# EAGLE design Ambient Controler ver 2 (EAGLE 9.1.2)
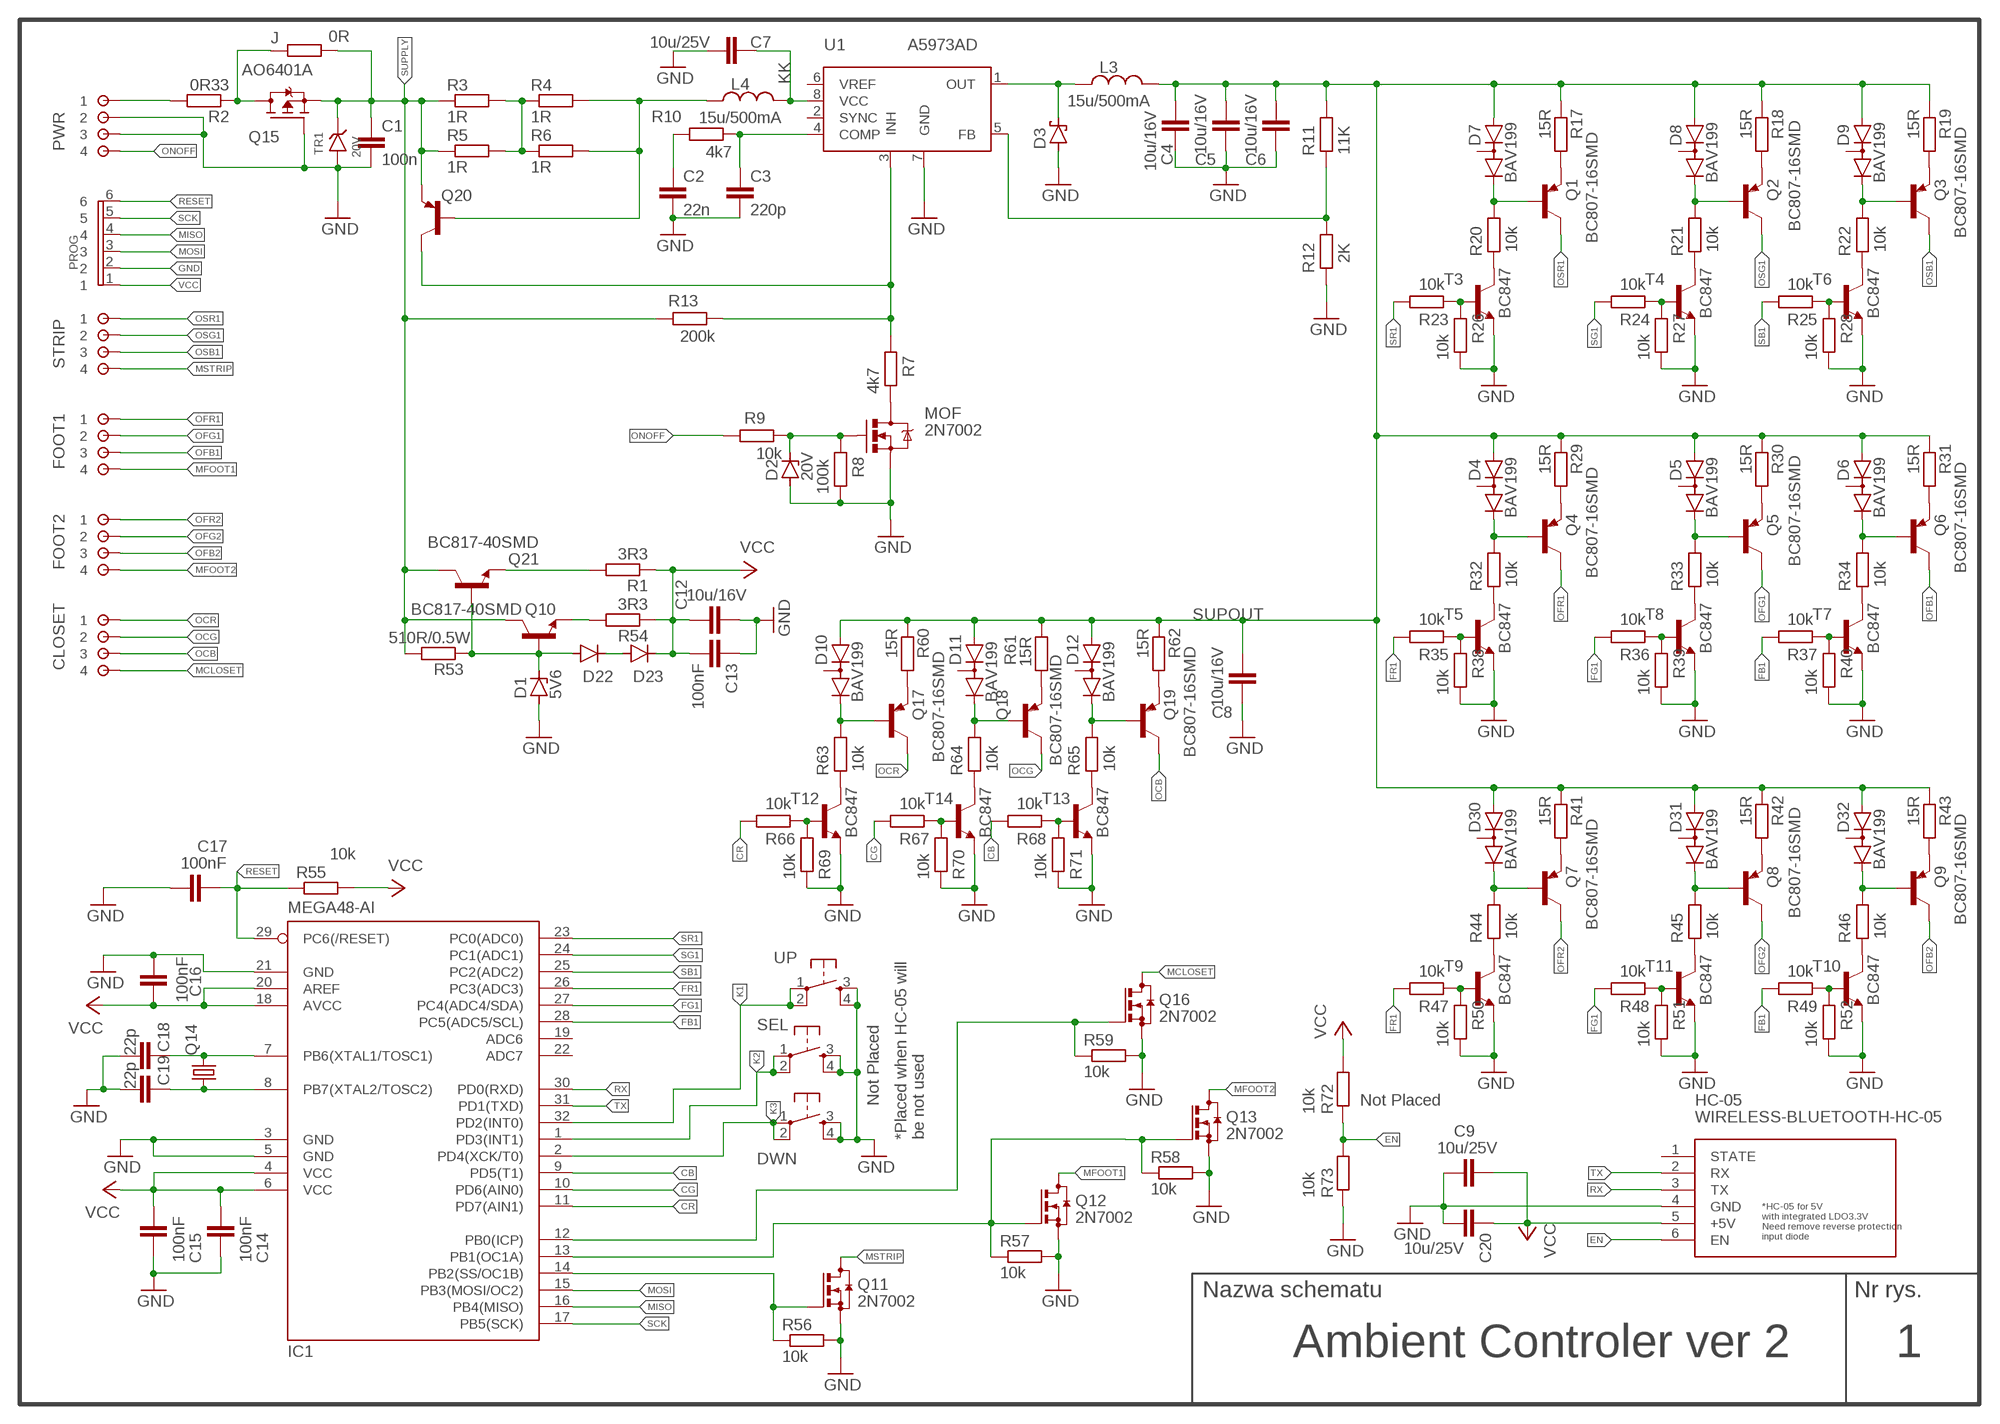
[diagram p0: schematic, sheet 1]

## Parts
C1  100n  C-EUC0805  [C0805]
C2  22n  C-EUC0805  [C0805]
C3  220p  C-EUC0805  [C0805]
C4  10u/16V  C-EUC1206  [C1206]
C5  10u/16V  C-EUC1206  [C1206]
C6  10u/16V  C-EUC1206  [C1206]
C7  10u/25V  C-EUC1206  [C1206]
C8  10u/16V  C-EUC1206  [C1206]
C9  10u/25V  C-EUC1206  [C1206]
C12  10u/16V  C-EUC1206  [C1206]
C13  100nF  C-EUC0805  [C0805]
C14  100nF  C-EUC0805  [C0805]
C15  100nF  C-EUC0805  [C0805]
C16  100nF  C-EUC0805  [C0805]
C17  100nF  C-EUC0805  [C0805]
C18  22p  C-EUC0805  [C0805]
C19  22p  C-EUC0805  [C0805]
C20  10u/25V  C-EUC1206  [C1206]
CLOSET  ARK254-4  [ARK254-4]
D1  5V6  ZENER-DIODESOD80C  [SOD80C]
D2  20V  ZENER-DIODESOD80C  [SOD80C]
D3  SCHOTTKY-DIODESMD  [SMB]
D4  BAV199  [SOT23]
D5  BAV199  [SOT23]
D6  BAV199  [SOT23]
D7  BAV199  [SOT23]
D8  BAV199  [SOT23]
D9  BAV199  [SOT23]
D10  BAV199  [SOT23]
D11  BAV199  [SOT23]
D12  BAV199  [SOT23]
D22  DIODE-MINIMELF  [MINIMELF]
D23  DIODE-MINIMELF  [MINIMELF]
D30  BAV199  [SOT23]
D31  BAV199  [SOT23]
D32  BAV199  [SOT23]
DWN  uSW  DTSM-6  [DTSM-6]
FOOT1  ARK254-4  [ARK254-4]
FOOT2  ARK254-4  [ARK254-4]
HC-05  WIRELESS-BLUETOOTH-HC-05  [WIRELESS-BLUETOOTH-HC-05]
IC1  MEGA48-AI  MEGA8-AI  [TQFP32-08]
J  0R  R-EU_R1206  [R1206]
L3  15u/500mA  L_MOLDED-1812(4532-METRIC)  [INDM4532X340]
L4  15u/500mA  L_MOLDED-1812(4532-METRIC)  [INDM4532X340]
MOF  2N7002  AO3442  [AO3442]
PROG  GOLDPIN6  [GOLDPIN6]
PWR  ARK254-4  [ARK254-4]
Q1  BC807-16SMD  [SOT23-BEC]
Q2  BC807-16SMD  [SOT23-BEC]
Q3  BC807-16SMD  [SOT23-BEC]
Q4  BC807-16SMD  [SOT23-BEC]
Q5  BC807-16SMD  [SOT23-BEC]
Q6  BC807-16SMD  [SOT23-BEC]
Q7  BC807-16SMD  [SOT23-BEC]
Q8  BC807-16SMD  [SOT23-BEC]
Q9  BC807-16SMD  [SOT23-BEC]
Q10  BC817-40SMD  [SOT23-BEC]
Q11  2N7002  BSS123  [SOT23]
Q12  2N7002  BSS123  [SOT23]
Q13  2N7002  BSS123  [SOT23]
Q14  CRYSTALHC49S  [HC49/S]
Q15  AO6401A  BSL307SP  [SC74_INFINEON]
Q16  2N7002  BSS123  [SOT23]
Q17  BC807-16SMD  [SOT23-BEC]
Q18  BC807-16SMD  [SOT23-BEC]
Q19  BC807-16SMD  [SOT23-BEC]
Q20  BC807-16SMD  [SOT23-BEC]
Q21  BC817-40SMD  [SOT23-BEC]
R1  3R3  R-EU_M0805  [M0805]
R2  0R33  R-EU_R1206  [R1206]
R3  1R  R-EU_R1206  [R1206]
R4  1R  R-EU_R1206  [R1206]
R5  1R  R-EU_R1206  [R1206]
R6  1R  R-EU_R1206  [R1206]
R7  4k7  R-EU_R0805  [R0805]
R8  100k  R-EU_R0805  [R0805]
R9  10k  R-EU_R0805  [R0805]
R10  4k7  R-EU_R0805  [R0805]
R11  11K  R-EU_R0805  [R0805]
R12  2K  R-EU_R0805  [R0805]
R13  200k  R-EU_R0805  [R0805]
R17  15R  R-EU_R0805  [R0805]
R18  15R  R-EU_R0805  [R0805]
R19  15R  R-EU_R0805  [R0805]
R20  10k  R-EU_R0805  [R0805]
R21  10k  R-EU_R0805  [R0805]
R22  10k  R-EU_R0805  [R0805]
R23  10k  R-EU_R0805  [R0805]
R24  10k  R-EU_R0805  [R0805]
R25  10k  R-EU_R0805  [R0805]
R26  10k  R-EU_R0805  [R0805]
R27  10k  R-EU_R0805  [R0805]
R28  10k  R-EU_R0805  [R0805]
R29  15R  R-EU_R0805  [R0805]
R30  15R  R-EU_R0805  [R0805]
R31  15R  R-EU_R0805  [R0805]
R32  10k  R-EU_R0805  [R0805]
R33  10k  R-EU_R0805  [R0805]
R34  10k  R-EU_R0805  [R0805]
R35  10k  R-EU_R0805  [R0805]
R36  10k  R-EU_R0805  [R0805]
R37  10k  R-EU_R0805  [R0805]
R38  10k  R-EU_R0805  [R0805]
R39  10k  R-EU_R0805  [R0805]
R40  10k  R-EU_R0805  [R0805]
R41  15R  R-EU_R0805  [R0805]
R42  15R  R-EU_R0805  [R0805]
R43  15R  R-EU_R0805  [R0805]
R44  10k  R-EU_R0805  [R0805]
R45  10k  R-EU_R0805  [R0805]
R46  10k  R-EU_R0805  [R0805]
R47  10k  R-EU_R0805  [R0805]
R48  10k  R-EU_R0805  [R0805]
R49  10k  R-EU_R0805  [R0805]
R50  10k  R-EU_R0805  [R0805]
R51  10k  R-EU_R0805  [R0805]
R52  10k  R-EU_R0805  [R0805]
R53  510R/0.5W  R-EU_R1206  [R1206]
R54  3R3  R-EU_M0805  [M0805]
R55  10k  R-EU_M0805  [M0805]
R56  10k  R-EU_M0805  [M0805]
R57  10k  R-EU_M0805  [M0805]
R58  10k  R-EU_M0805  [M0805]
R59  10k  R-EU_M0805  [M0805]
R60  15R  R-EU_R0805  [R0805]
R61  15R  R-EU_R0805  [R0805]
R62  15R  R-EU_R0805  [R0805]
R63  10k  R-EU_R0805  [R0805]
R64  10k  R-EU_R0805  [R0805]
R65  10k  R-EU_R0805  [R0805]
R66  10k  R-EU_R0805  [R0805]
R67  10k  R-EU_R0805  [R0805]
R68  10k  R-EU_R0805  [R0805]
R69  10k  R-EU_R0805  [R0805]
R70  10k  R-EU_R0805  [R0805]
R71  10k  R-EU_R0805  [R0805]
R72  10k  R-EU_M0805  [M0805]
R73  10k  R-EU_M0805  [M0805]
SEL  SEL  DTSM-6  [DTSM-6]
STRIP  ARK254-4  [ARK254-4]
T3  BC847  [SOT23]
T4  BC847  [SOT23]
T5  BC847  [SOT23]
T6  BC847  [SOT23]
T7  BC847  [SOT23]
T8  BC847  [SOT23]
T9  BC847  [SOT23]
T10  BC847  [SOT23]
T11  BC847  [SOT23]
T12  BC847  [SOT23]
T13  BC847  [SOT23]
T14  BC847  [SOT23]
TR1  20V  TRANSIL  [DO214AC_MONODIR]
U1  A5973AD  L5973D  [HSOP8]
UP  NOT_PLACED  DTSM-6  [DTSM-6]

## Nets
CB: IC1.9(PD5(T1)) R68.1
CG: IC1.10(PD6(AIN0)) R67.1
CR: IC1.11(PD7(AIN1)) R66.1
EN: HC-05.6(EN) R72.1 R73.2
FB1: IC1.28(PC5(ADC5/SCL)) R37.1 R49.1
FG1: IC1.27(PC4(ADC4/SDA)) R36.1 R48.1
FR1: IC1.26(PC3(ADC3)) R35.1 R47.1
GND: C1.2 C2.2 C3.2 C4.1 C5.1 C6.1 C7.2 C8.1 C9.2 C12.2 C13.1 C14.1 C15.1 C16.2 C17.2 C18.2 C19.2 C20.2 D1.A D2.A D3.A DWN.3 DWN.4 HC-05.4(GND) IC1.3(GND) IC1.5(GND) IC1.21(GND) MOF.2(S) PROG.2 PWR.2 PWR.3 Q11.2(S) Q12.2(S) Q13.2(S) Q15.3(G) Q16.2(S) R8.1 R12.2 R26.1 R27.1 R28.1 R38.1 R39.1 R40.1 R50.1 R51.1 R52.1 R56.2 R57.2 R58.2 R59.2 R69.1 R70.1 R71.1 R73.1 SEL.3 SEL.4 T3.2(E) T4.2(E) T5.2(E) T6.2(E) T7.2(E) T8.2(E) T9.2(E) T10.2(E) T11.2(E) T12.2(E) T13.2(E) T14.2(E) TR1.P$1 U1.7(GND) UP.3 UP.4
K1: IC1.32(PD2(INT0)) UP.1 UP.2
K2: IC1.1(PD3(INT1)) SEL.1 SEL.2
K3: DWN.1 DWN.2 IC1.2(PD4(XCK/T0))
KK: C7.1 L4.2 U1.8(VCC)
MCLOSET: CLOSET.4 Q16.3(D)
MFOOT1: FOOT1.4 Q12.3(D)
MFOOT2: FOOT2.4 Q13.3(D)
MISO: IC1.16(PB4(MISO)) PROG.4
MOSI: IC1.15(PB3(MOSI/OC2)) PROG.3
MSTRIP: Q11.3(D) STRIP.4
N$1: J.2 Q15.1(D) Q15.2(D) Q15.5(D) Q15.6(D) R2.1
N$3: Q21.E R1.2
N$4: Q20.C R7.2 R13.1 U1.3(INH)
N$5: R3.2 R4.1 R5.2 R6.1
N$6: Q1.E R17.2
N$7: MOF.3(D) R7.1
N$8: PWR.1 R2.2
N$9: C2.1 R10.2
N$10: D7.2(C) Q1.B R20.1
N$11: C3.1 R10.1 U1.4(COMP)
N$12: L4.1 Q20.B R4.2 R6.2
N$13: D2.C MOF.1(G) R8.2 R9.1
N$16: D1.C D22.A Q10.B Q21.B R53.1
N$19: R11.2 R12.1 U1.5(FB)
N$21: Q2.E R18.2
N$23: Q3.E R19.2
N$24: D8.2(C) Q2.B R21.1
N$25: D9.2(C) Q3.B R22.1
N$26: R20.2 T3.3(C)
N$27: R21.2 T4.3(C)
N$29: R23.2 R26.2 T3.1(B)
N$30: R22.2 T6.3(C)
N$31: R24.2 R27.2 T4.1(B)
N$32: R25.2 R28.2 T6.1(B)
N$33: Q4.E R29.2
N$35: D22.C D23.A
N$37: Q5.E R30.2
N$39: Q6.E R31.2
N$40: D4.2(C) Q4.B R32.1
N$41: D5.2(C) Q5.B R33.1
N$42: D6.2(C) Q6.B R34.1
N$43: R32.2 T5.3(C)
N$44: R34.2 T7.3(C)
N$45: R33.2 T8.3(C)
N$46: R35.2 R38.2 T5.1(B)
N$47: R36.2 R39.2 T8.1(B)
N$48: R37.2 R40.2 T7.1(B)
N$49: Q7.E R41.2
N$51: Q10.E R54.2
N$53: Q8.E R42.2
N$55: Q9.E R43.2
N$56: D30.2(C) Q7.B R44.1
N$57: D31.2(C) Q8.B R45.1
N$58: D32.2(C) Q9.B R46.1
N$59: R44.2 T9.3(C)
N$60: R46.2 T10.3(C)
N$61: R45.2 T11.3(C)
N$62: R47.2 R50.2 T9.1(B)
N$63: R48.2 R51.2 T11.1(B)
N$64: R49.2 R52.2 T10.1(B)
N$65: IC1.14(PB2(SS/OC1B)) Q11.1(G) R56.1
N$67: IC1.13(PB1(OC1A)) Q12.1(G) Q13.1(G) R57.1 R58.1
N$71: IC1.12(PB0(ICP)) Q16.1(G) R59.1
N$72: Q17.E R60.2
N$75: Q18.E R61.2
N$77: Q19.E R62.2
N$78: C18.1 IC1.7(PB6(XTAL1/TOSC1)) Q14.2
N$79: C19.1 IC1.8(PB7(XTAL2/TOSC2)) Q14.1
N$80: D10.2(C) Q17.B R63.1
N$81: D11.2(C) Q18.B R64.1
N$82: D12.2(C) Q19.B R65.1
N$83: R63.2 T12.3(C)
N$84: R65.2 T13.3(C)
N$85: R64.2 T14.3(C)
N$87: R66.2 R69.2 T12.1(B)
N$88: R67.2 R70.2 T14.1(B)
N$89: R68.2 R71.2 T13.1(B)
OCB: CLOSET.3 Q19.C
OCG: CLOSET.2 Q18.C
OCR: CLOSET.1 Q17.C
OFB1: FOOT1.3 Q6.C
OFB2: FOOT2.3 Q9.C
OFG1: FOOT1.2 Q5.C
OFG2: FOOT2.2 Q8.C
OFR1: FOOT1.1 Q4.C
OFR2: FOOT2.1 Q7.C
ONOFF: PWR.4 R9.2
OSB1: Q3.C STRIP.3
OSG1: Q2.C STRIP.2
OSR1: Q1.C STRIP.1
OUT: D3.C L3.1 U1.1(OUT)
RESET: C17.1 IC1.29(PC6(/RESET)) PROG.6 R55.1
RX: HC-05.3(TX) IC1.30(PD0(RXD))
SB1: IC1.25(PC2(ADC2)) R25.1
SCK: IC1.17(PB5(SCK)) PROG.5
SG1: IC1.24(PC1(ADC1)) R24.1
SR1: IC1.23(PC0(ADC0)) R23.1
SUPOUT: C4.2 C5.2 C6.2 C8.2 D4.1(A) D5.1(A) D6.1(A) D7.1(A) D8.1(A) D9.1(A) D10.1(A) D11.1(A) D12.1(A) D30.1(A) D31.1(A) D32.1(A) L3.2 R11.1 R17.1 R18.1 R19.1 R29.1 R30.1 R31.1 R41.1 R42.1 R43.1 R60.1 R61.1 R62.1
SUPPLY: C1.1 J.1 Q10.C Q15.4(S) Q20.E Q21.C R3.1 R5.1 R13.2 R53.2 TR1.P$2
TX: HC-05.2(RX) IC1.31(PD1(TXD))
VCC: C9.1 C12.1 C13.2 C14.2 C15.2 C16.1 C20.1 D23.C HC-05.5(+5V) IC1.4(VCC) IC1.6(VCC) IC1.18(AVCC) IC1.20(AREF) PROG.1 R1.1 R54.1 R55.2 R72.2
Unconnected: D4.3(AC) D5.3(AC) D6.3(AC) D7.3(AC) D8.3(AC) D9.3(AC) D10.3(AC) D11.3(AC) D12.3(AC) D30.3(AC) D31.3(AC) D32.3(AC) HC-05.1(STATE) IC1.19(ADC6) IC1.22(ADC7) U1.2(SYNC) U1.6(VREF)

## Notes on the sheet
- Not Placed | Not Placed
- *Placed when HC-05 will
  be not used
- *HC-05 for 5V 
  with integrated LDO3.3V
  Need remove reverse protection
  input diode
- Ambient Controler ver 2 | 1

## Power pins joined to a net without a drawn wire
GND: U1.9(GND)

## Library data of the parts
C1-C9 C12-C20 = rcl:C-EU: CAPACITOR, European symbol; SPICEPREFIX: C
CLOSET FOOT1 FOOT2 PWR STRIP = ark254:ARK254-4
D1 D2 = diode:ZENER-DIODE: Z-Diode
D3 = diode:SCHOTTKY-DIODE: Schottky Diode
D4-D12 D30-D32 = diode:BAV199: DIODE low-leakage double diode
D22 D23 = diode:DIODE-: DIODE
DWN SEL UP = switch-tact:DTSM-6
HC-05 = diy-modules:WIRELESS-BLUETOOTH-HC-05: Bluetooth Transceiver Module based on HC-05 board Tutorial is available here: https://arduino-info.wikispaces.com/BlueTooth-HC05-HC06-Modules-How-To Click here to find device on ebay.com
IC1 = atmel:MEGA8: MICROCONTROLLER 8 Kbytes FLASH, 1 kbytes SRAM, 512 bytes EEPROM, USART, 6-channel 10 bit ADC, 2-channel 8 bit ADC Pin compatible with Atmega48, ATMega88, ATMega168 Source: avr.lbr; MPN: ATMEGA8-16AU; OC_FARNELL: 9171371; OC_NEWARK: 73M8863
J R1-R13 R17-R73 = rcl:R-EU_: RESISTOR, European symbol; SPICEPREFIX: R
L3 L4 = Inductor:L: Inductor Fixed - Generic; CATEGORY: Inductor; SUB-CATEGORY: Fixed
MOF = AO3442:AO3442
PROG = GOLDPIN6:GOLDPIN6
Q1-Q9 Q17-Q19 = transistor-pnp:BC807*: PNP Transistror
Q10 Q21 = transistor-npn:BC817*: NPN Transistor
Q11-Q13 Q16 = transistor-small-signal:BSS123: N-CHANNEL MOS FET
Q14 = crystal:CRYSTAL: CRYSTAL; OC_FARNELL: 1667008; OC_NEWARK: unknown
Q15 = transistor-fet:BSL307SP: OptiMOS(R)-P Small-Signal-Transistor P-Channel, Enhancement mode, Logic Level ID -5.5 A Source: http://www.infineon.com/upload/Document/BSL307SP_Rev%201.2.pdf
Q20 = transistor-pnp:BC807*: PNP Transistror; SPICEPREFIX: Q
T3-T14 = transistor-neu-to92:BC847: NPN TRANSISTOR
TR1 = transil2:TRANSIL
U1 = l5973d:L5973D: 2.5A switch step down switching regulator

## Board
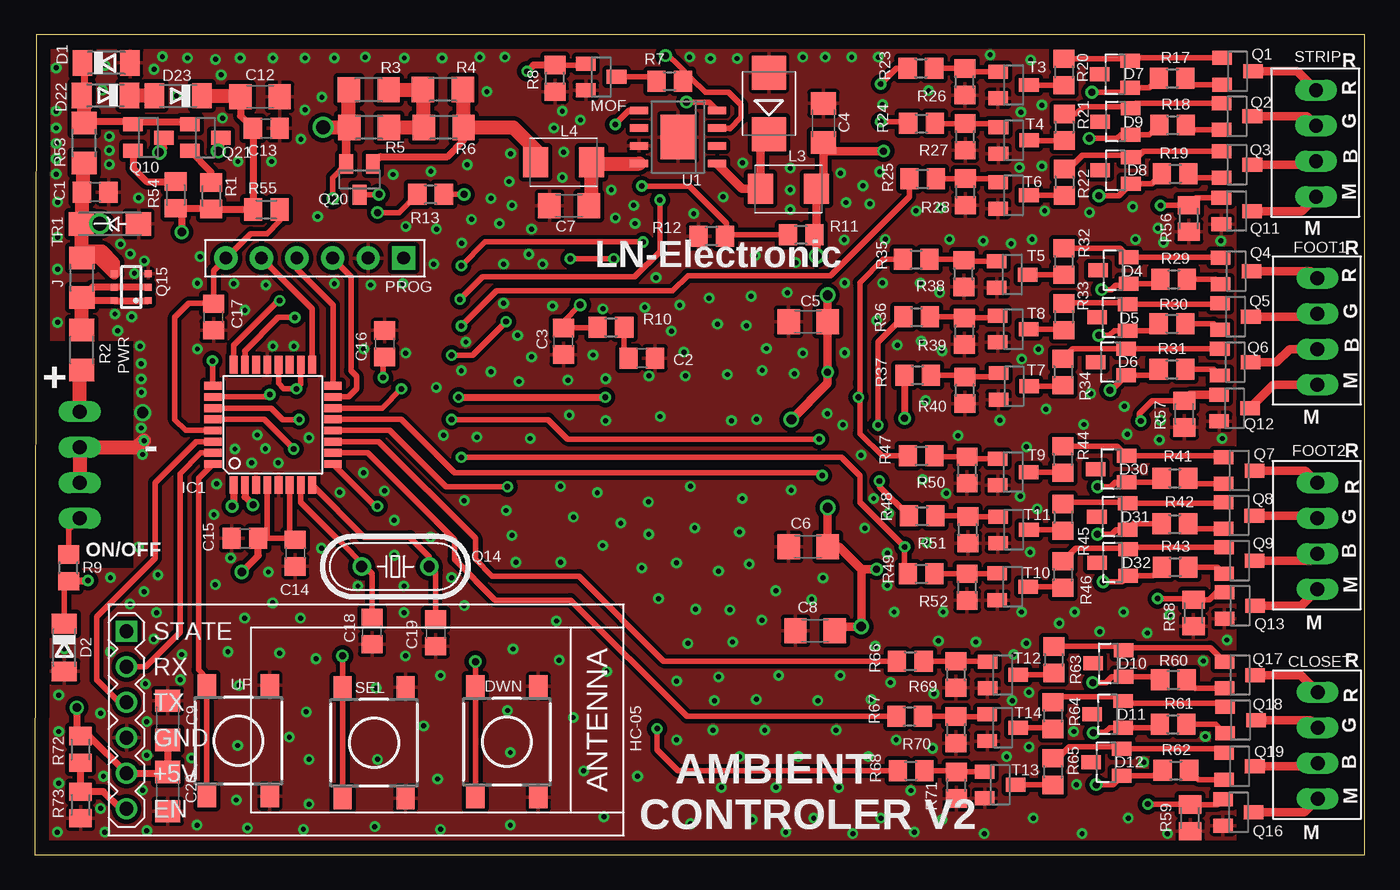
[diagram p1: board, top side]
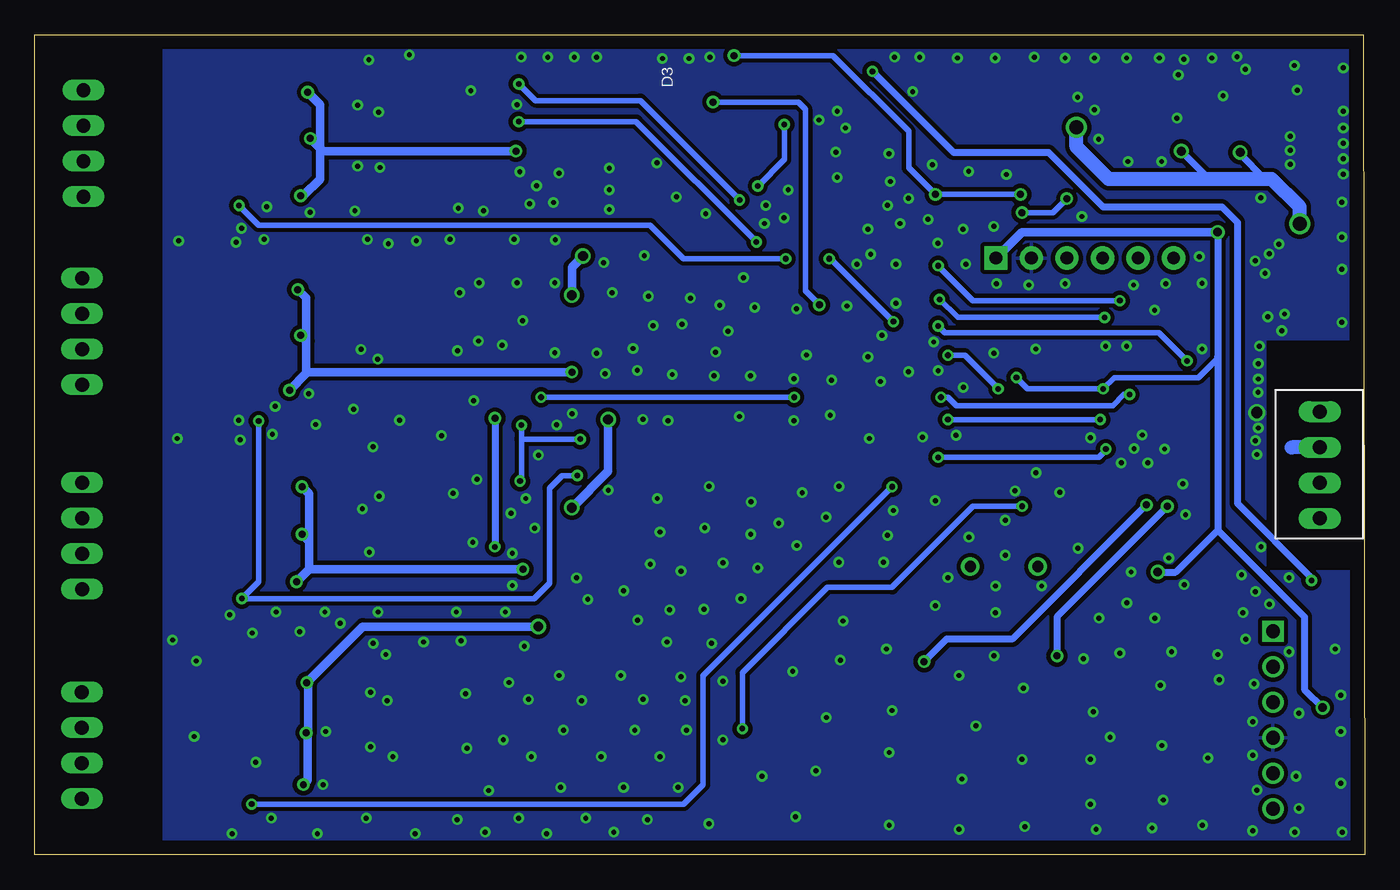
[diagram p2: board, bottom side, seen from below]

Size 95.1 x 58.6 mm. Coordinates in mm from the lower left corner, seen from the top.
Outline: 0,0 95.1,0 95.1,58.6 0.1,58.6 0,0
Copper layers (1*16): Top 0.035mm / dielectric 1.5mm / Bottom 0.035mm
Design rules "default *": minimum track width 6mil, minimum drill 0.35mm, track to track 6mil, track to pad 6mil, pad to pad 6mil, via to via 6mil, smd to smd 6mil, copper to edge 40mil, drill to drill 6mil, minimum pad ring 10mil, minimum via ring 8mil, stop-mask expansion 4mil, vias tented up to drill 30mil, thermal gap 10mil

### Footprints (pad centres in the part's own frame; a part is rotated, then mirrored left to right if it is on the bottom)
C0805 = smd 1.3 x 1.5: 1 -0.95,0; 2 0.95,0
C1206 = smd 1.6 x 1.8: 1 -1.4,0; 2 1.4,0
ARK254-4 = drill 1 long: 1 -0.06,0; 2 2.48,0; 3 5.02,0; 4 7.56,0
SOD80C = smd 1.4 x 1.8: A 1.7,0; C -1.7,0
SMB = smd 2.4 x 2.4: A 2.2,0; C -2.2,0
SOT23 = smd 1 x 1.4: 1 -0.95,-1.1; 2 0.95,-1.1; 3 0,1.1
MINIMELF = smd 1.4 x 1.8: A 1.7,0; C -1.7,0
DTSM-6 = smd 1.55 x 1.3: 1 -3.975,2.25; 2 3.975,2.25; 3 -3.975,-2.25; 4 3.975,-2.25
WIRELESS-BLUETOOTH-HC-05 = drill 1 square: 1 -6.35,-17.145 | drill 1: 2 -3.81,-17.145; 3 -1.27,-17.145; 4 1.27,-17.145; 5 3.81,-17.145; 6 6.35,-17.145
TQFP32-08 = smd 1.27 x 0.559: 1 -4.293,2.8; 2 -4.293,2; 3 -4.293,1.2; 4 -4.293,0.4; 5 -4.293,-0.4; 6 -4.293,-1.2; 7 -4.293,-2; 8 -4.293,-2.8; 17 4.293,-2.8; 18 4.293,-2; 19 4.293,-1.2; 20 4.293,-0.4; 21 4.293,0.4; 22 4.293,1.2; 23 4.293,2; 24 4.293,2.8 | smd 0.559 x 1.27: 9 -2.8,-4.293; 10 -2,-4.293; 11 -1.2,-4.293; 12 -0.4,-4.293; 13 0.4,-4.293; 14 1.2,-4.293; 15 2,-4.293; 16 2.8,-4.293; 25 2.8,4.293; 26 2,4.293; 27 1.2,4.293; 28 0.4,4.293; 29 -0.4,4.293; 30 -1.2,4.293; 31 -2,4.293; 32 -2.8,4.293
R1206 = smd 1.6 x 1.803: 1 -1.422,0; 2 1.422,0
INDM4532X340 = smd 1.793 x 2.129: 1 -2.009,0; 2 2.009,0
AO3442 = smd 1 x 1.4: 1 -0.95,-1.1; 2 0.95,-1.1; 3 0,1.1
GOLDPIN6 = drill 0.9 pad 1.676 square: 1 0,0 | drill 0.9 pad 1.676: 2 2.54,0; 3 5.08,0; 4 7.62,0; 5 10.16,0; 6 12.7,0
SOT23-BEC = smd 1 x 1.4: B -0.95,-1.1; C 0,1.1; E 0.95,-1.1
HC49/S = drill 0.813: 1 -2.413,0; 2 2.413,0
SC74_INFINEON = smd 0.5 x 0.5: 1 -0.95,-1.2; 2 0,-1.2; 3 0.95,-1.2; 4 0.95,1.2; 5 0,1.2; 6 -0.95,1.2
M0805 = smd 1.3 x 1.6: 1 -0.95,0; 2 0.95,0
R0805 = smd 1.3 x 1.5: 1 -0.95,0; 2 0.95,0
DO214AC_MONODIR = smd 1.8 x 1.7: P$1 -2.05,0; P$2 2.05,0
HSOP8 = smd 0.54 x 1.27: 1 -1.905,-2.785; 2 -0.635,-2.785; 3 0.635,-2.785; 4 1.905,-2.785; 5 1.905,2.785; 6 0.635,2.785; 7 -0.635,2.785; 8 -1.905,2.785 | smd 3.2 x 2.51: 9 0,0

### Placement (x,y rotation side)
C1  4.31,47.36 0 top
C2  43.4,35.5 0 top
C3  37.8,36.7 270 top
C4  56.4,52.3 270 top
C5  55.3,38.1 0 top
C6  55.3,22 0 top
C7  38.2,46.4 180 top
C8  55.8,16 0 top
C9  9.5,9.6 90 top
C12  16.1,54.17 0 top
C13  16.54,51.92 180 top
C14  18.62,21.55 90 top
C15  15.02,22.61 0 top
C16  25.02,36.52 90 top
C17  12.78,38.43 270 top
C18  24.11,15.99 270 top
C19  28.66,15.85 270 top
C20  9.5,4.5 270 top
CLOSET  91.75,11.55 270 top
D1  5.1,56.6 0 top
D2  2.1,14.8 270 top
D3  52.5,53.7 90 top
D4  77.13,41.77 90 top
D5  77.06,38.41 90 top
D6  76.95,35.21 90 top
D7  77.24,55.79 90 top
D8  77.28,52.41 90 top
D9  77.28,48.92 90 top
D10  76.78,13.66 90 top
D11  76.73,10.03 90 top
D12  76.63,6.6 90 top
D22  5.05,54.28 180 top
D23  10.24,54.25 180 top
D30  76.97,27.56 90 top
D31  77.05,24.16 90 top
D32  77.08,20.88 90 top
DWN  33.75,8.06 90 top
FOOT1  91.73,41.16 270 top
FOOT2  91.73,26.53 270 top
HC-05  23.69,9.62 270 top
IC1  17.02,30.72 90 top
J  3.36,41.24 270 top
L3  53.9,47.6 0 top
L4  37.8,49.5 0 top
MOF  40.5,55.6 270 top
PROG  26.37,42.64 180 top
PWR  3.2,31.6 270 bottom
Q1  86.01,56 270 top
Q2  85.97,52.78 270 top
Q3  85.97,49.33 270 top
Q4  85.91,41.71 270 top
Q5  85.87,38.46 270 top
Q6  85.85,35.2 270 top
Q7  86.13,27.45 270 top
Q8  86.12,24.24 270 top
Q9  86.14,21.01 270 top
Q10  8.12,51.26 270 top
Q11  85.95,46.01 270 top
Q12  85.8,31.92 270 top
Q13  86.18,17.8 270 top
Q14  25.78,20.59 180 top
Q15  6.89,40.56 90 top
Q16  86.07,3.02 270 top
Q17  86.18,12.83 270 top
Q18  86.23,9.62 270 top
Q19  86.15,6.31 270 top
Q20  23.22,48.28 180 top
Q21  12.19,51.26 270 top
R1  12.6,47.1 90 top
R2  3.34,36.07 270 top
R3  23.87,54.69 0 top
R4  29.18,54.7 0 top
R5  23.9,51.98 0 top
R6  29.24,51.98 0 top
R7  45.4,55.3 0 top
R8  37.2,55.5 90 top
R9  2.4,20.5 90 top
R10  41.2,37.7 0 top
R11  54.8,44.3 180 top
R12  48.4,44.2 180 top
R13  28.3,47.2 180 top
R17  81.33,55.51 0 top
R18  81.38,52.16 0 top
R19  81.55,48.67 0 top
R20  73.59,55.95 270 top
R21  73.62,52 270 top
R22  73.63,48.07 270 top
R23  63.37,56.23 0 top
R24  63.41,52.28 0 top
R25  63.49,48.32 0 top
R26  66.5,55.26 90 top
R27  66.53,51.32 90 top
R28  66.55,47.38 90 top
R29  81.45,41.14 0 top
R30  81.32,37.96 0 top
R31  81.32,34.69 0 top
R32  73.58,42.4 270 top
R33  73.59,38.45 270 top
R34  73.54,34.51 270 top
R35  63.03,42.55 0 top
R36  63.06,38.44 0 top
R37  63.13,34.28 0 top
R38  66.43,41.53 90 top
R39  66.49,37.42 90 top
R40  66.52,33.2 90 top
R41  81.53,26.91 0 top
R42  81.53,23.64 0 top
R43  81.55,20.55 0 top
R44  73.51,28.25 270 top
R45  73.54,24.11 270 top
R46  73.51,20.02 270 top
R47  63.39,28.51 0 top
R48  63.45,24.21 0 top
R49  63.39,20.08 0 top
R50  66.68,27.49 90 top
R51  66.73,23.22 90 top
R52  66.68,19.12 90 top
R53  3.52,50.88 270 top
R54  10.07,47.17 90 top
R55  16.56,46.12 180 top
R56  82.54,45.47 270 top
R57  82.21,31.49 270 top
R58  82.87,17.26 270 top
R59  82.63,2.62 270 top
R60  81.42,12.49 0 top
R61  81.4,9.32 0 top
R62  81.6,6.01 0 top
R63  72.86,13.93 270 top
R64  72.8,9.93 270 top
R65  72.8,5.93 270 top
R66  62.61,13.83 0 top
R67  62.56,9.88 0 top
R68  62.66,5.99 0 top
R69  65.89,12.87 90 top
R70  65.88,8.91 90 top
R71  65.91,4.95 90 top
R72  3.25,7.52 90 top
R73  3.26,3.55 90 top
SEL  24.25,8 90 top
STRIP  91.63,54.6 270 top
T3  69.99,55.02 270 top
T4  70.01,51.07 270 top
T5  69.9,41.47 270 top
T6  69.99,47.13 270 top
T7  70.02,33.48 270 top
T8  69.97,37.56 270 top
T9  69.96,27.35 270 top
T10  69.93,19.15 270 top
T11  69.99,23.22 270 top
T12  69.23,12.84 270 top
T13  69.04,4.98 270 top
T14  69.22,9.07 270 top
TR1  5.36,45.09 180 top
U1  46,51.3 90 top
UP  14.55,8.14 90 top

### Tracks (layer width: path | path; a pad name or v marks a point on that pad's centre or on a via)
CB  (via drill 0.4)
  Top 0.406: IC1.9 24.33,24.9 v24.5,24.9 | R68.1 46.01,5.99 44.5,7.5 v44.5,9
  Bottom 0.406: v24.5,24.9 28,24.9 33.8,19.1 38.4,19.1 44.5,13 v44.5,9
CG
  Top 0.406: IC1.10 23.78,28.72 30,22.5 30,21.1 32.9,18.2 38.3,18.2 46.62,9.88 R67.1
CR
  Top 0.406: IC1.11 24.58,29.52 31.5,22.6 31.5,21.1 32.7,19.9 38.9,19.9 44.97,13.83 R66.1
EN
  Top 0.508: R72.1 R73.2 4.9,4.5 6.13,3.27 HC-05.6
FB1  (via drill 0.4, 0.5)
  Top 0.406: 62.2,20.32 v62.2,22 59,25.2 59,27.1 57.7,28.4 41.6,28.4 v30.5,28.4 | IC1.28 16.38,31.12 v18.5,29
  Top 0.508: R37.1 62.18,31.22 v62.2,31.2 | 62.2,20.32 R49.1
  Bottom 0.406: 18.5,28.9 19,28.4 v30.5,28.4
  Bottom 0.508: v62.2,31.2 v62.2,22 | v18.5,29 18.5,28.9
FG1  (via drill 0.4)
  Top 0.406: R36.1 60.3,36.62 v60.3,30.7 | v60.4,26.7 60.4,26.31 R48.1 | IC1.27 16.88,31.92 17.7,31.1 v18.9,31.1 | v29.8,31.1 36.7,31.1 38.1,29.7 v56.1,29.7
  Top 0.508: v60.3,30.7 60.3,30.5 v60.3,30.7
  Bottom 0.406: v60.3,30.7 60.3,29.7 | 60.3,29.7 60.3,26.8 | v18.9,31.1 v29.8,31.1 | v56.1,29.7 60.3,29.7
  Bottom 0.508: 60.3,26.8 v60.4,26.7
FR1  (via drill 0.4)
  Top 0.406: R35.1 60.65,42.55 59,40.9 59,33.7 59,32.7 | R47.1 60.6,28.5 59,30.1 59,32.7 | IC1.26 16.62,32.72 v16.8,32.9 | v58.9,32.7 59,32.7
  Top 0.508: R47.1 | v30.3,32.7 v40.8,32.7
  Bottom 0.406: v16.8,32.9 17.2,32.9 18,32.1 29.2,32.1 29.8,32.7 v30.3,32.7 | v40.8,32.7 v58.9,32.7
GND  (via drill 0.35, 0.8)
  Top 1.016: PWR.3 PWR.2 7.32,29.12 v7.8,29.6
  Bottom 1.016: PWR.2 5.22,29.12
  other vias: 7.7,31.6 43.9,22.9 33.8,10.3 17,18 5.4,19.8 7.4,22 2.1,14.7 1.7,11.4 4.7,10.1 1.7,5.1 1.7,8.8 1.6,1.6 5,1.6 4.7,3.3 4.9,5.6 5.4,14.5 6.8,17.9 7.8,18.8 8.8,20 8.7,17.3 8.5,15.4 8,1.7 7.7,4.6 8,7.1 8,9.5 7.9,12.2 10.5,14.3 10.4,12.5 11.2,6.9 18.2,8.4 11.6,2.1 14.4,3.9 14.5,7.8 14.6,12.1 13.8,14.5 15,16.9 19,16.9 20.1,14 17.5,14.4 19.4,10.2 19.6,6.8 19.6,3.6 19.2,1.8 15.2,1.9 24.3,2 24.5,6.8 24.4,11.9 27.8,9.2 28.8,5.4 29,1.8 34,2.1 34,7.3 34.2,14.7 30.7,17.8 37.3,16.7 40.9,13.1 38.5,9.8 43.1,5.6 40.7,2.7 46.9,2.2 29,12.8 26.5,14.2 26.4,17.3 25.7,21.4 26.4,19.2 20.5,21.9 23.1,19.2 28.3,22.7 25.7,23.9 21.8,25.9 23.5,27.3 25,26 30.7,25.3 33.7,24.6 17.4,28 15.9,30 14.3,29 15.5,28 19.6,29.8 28.7,33.4 30.5,34.6 13,26.5 12.8,24.3 14,21.2 12.9,19.3 16.7,20.2 29.8,19.8 37.5,13.9 45.9,8.2 45.9,12.4 40.6,22.1 43.4,20.5 44.6,18.3 46.7,15.1 49.9,15.2 41.9,23.7 49.7,17.5 60.1,14.9 67.3,15.2 70.9,15.1 70,14.3 64.3,11.5 61.2,12.3 59.8,11.1 57.6,12.8 56,11 53.2,12.8 51.6,11.1 48.9,12.7 48.6,11 48.5,8.9 50.4,7 52.2,8.9 54.6,7 57.3,8.9 59.6,7 61.6,8.2 64.2,7.6 49.1,4.8 53,4.8 57.5,4.8 62.65,4.58 51.3,2.5 55.7,2.6 60.5,2.6 64.9,2.5 58.5,1.5 53.7,1.6 62.9,1.6 67.9,1.5 71.4,2.6 74.9,1.5 78.2,2.6 81,1.5 69.5,7 71.1,7.7 69.9,11 71.1,11.6 74.3,8.8 74.5,5 79.3,6.6 83.71,8.44 83.56,13.84 85.26,15.34 81.16,17.14 79.56,15.84 77.86,17.34 76.16,15.94 74.36,17.34 73.26,16.54 70.56,17.34 64.96,17.34 61.46,17.34 47.26,17.54 55.56,18.24 60.96,19.24 60.96,21.54 59.36,23.34 61.05,24.4 59.99,25.46 59.09,28.56 47.19,23.36 54.09,26.06 52.99,18.86 51.09,20.76 50.39,23.06 48.89,20.26 45.89,20.86 50.59,25.46 51.99,16.76 56.36,19.78 43.88,25.22 46.88,26.32 37.58,26.32 40.82,31.02 38.22,31.42 38.12,33.92 40.82,34.02 34.62,33.82 43.92,34.22 46.52,34.22 44.72,31.32 49.52,34.32 48.82,37.92 43.62,39.12 34.12,22.82 51.22,39.92 39.92,35.72 40.62,39.02 32.62,34.52 34.52,37.12 33.52,39.42 33.52,42.22 35.32,42.92 36.32,42.22 26.32,40.82 24.02,40.72 21.42,40.82 16.52,40.72 14.22,40.82 15.02,38.92 26.52,44.92 5.02,56.42 58.02,46.62 20.22,45.62 25.62,48.62 31.22,45.42 30.52,43.72 28.52,42.22 28.72,44.72 33.22,45.12 35.52,44.72 42.92,45.12 42.82,46.42 41.22,47.52 41.52,45.52 54.02,46.12 39.02,52.52 34.12,46.42 34.02,50.12 33.92,48.12 47.12,45.82 30.92,49.32 31.82,57.02 49.22,47.02 33.62,57.02 54.92,57.02 58.42,57.02 52.02,34.62 37.02,39.22 45.52,37.42 38.52,24.12 54.02,47.52 57.62,48.72 60.42,48.82 59.72,46.52 23.62,57.02 56.52,57.02 60.32,57.02 60.62,53.62 63.92,54.62 63.02,46.02 64.82,46.22 70.42,49.12 72.02,49.22 72.22,46.02 75.42,45.92 78.52,46.32 71.22,56.82 68.32,57.18 70.52,53.08 72.02,53.58 84.82,43.88 80.72,43.78 80.32,44.78 78.72,43.98 71.32,43.98 69.82,43.68 67.82,43.88 65.42,43.98 60.82,43.98 53.82,40.18 54.32,34.38 52.32,36.18 48.22,39.78 40.22,25.88 54.02,49.08 57.92,35.88 35.52,35.58 46.12,39.28 60.22,38.18 60.62,40.88 63.32,40.88 64.72,40.18 46.42,35.92 61.68,36.42 64.88,36.02 63.38,36.72 70.58,35.42 71.78,36.12 56.68,31.52 57.78,30.72 63.48,26.82 65.18,25.82 70.48,25.62 71.68,24.72 16.48,29.02 7.62,33.05 31.62,29.85 35.42,29.75 7.52,36.35 54.92,35.85 5.92,37.45 5.72,38.65 6.92,38.45 6.12,43.65 57.88,43.95 37.12,51.95 11.62,40.85 11.82,42.75 16.92,49.55 26.42,56.95 29.12,56.95 19.32,56.95 19.32,53.25 20.52,54.15 14.68,56.95 21.42,56.95 17.02,56.95 12.92,56.85 9.12,57.05 10.92,56.95 8.52,56.15 4.82,54.65 10.12,54.25 1.52,56.25 1.52,53.15 5.32,51.35 28.32,48.85 1.62,41.85 1.62,38.05 11.62,36.15 17.02,36.35 18.52,36.35 23.52,36.15 26.52,35.85 30.82,36.65 44.42,41.25 63.72,32.45 66.02,29.95 69.02,31.05 70.92,29.15 72.32,31.85 75.02,30.75 77.92,32.05 78.12,30.05 75.52,32.95 50.88,37.82 63.78,22.32 71.18,21.62 34.4,20.9 37.6,20.9 49.82,31.02 51.62,31.12 39.25,5.98 32.62,46.92 7.82,42.45 7.12,41.55 80.52,31.05 80.42,29.65 84.92,29.75 50.22,56.92 48.32,56.92 46.82,57.02 37.82,50.22 37.72,48.42 7.6,30.5 7.7,28.6 7.6,34 7.6,35.1 6.82,42.95 1.62,44.15 1.62,46.65 7.42,46.95 19.02,51.15 32.32,54.55 37.72,53.15 50.62,49.45 59.22,47.82 51.52,42.82 54.42,42.32 57.92,40.88 29.22,29.98 64.62,15.28 14.52,49.55 13.42,52.65 5.32,49.35 1.52,51.95 1.52,50.85 1.52,49.75 1.52,48.65 5.32,50.35 13.32,55.75
  pour Bottom (isolate 0.305): 0.1,58.5 0.1,36.8 7.1,36.8 7.1,20.3 0.1,20.3 0.1,0.1 85.9,0.1 85.9,58.5
  pour Top (isolate 0.305): 0.1,58.5 0.1,36.8 7.1,36.8 7.1,20.4 0.1,20.4 0.1,0.1 85.9,0.1 85.9,58.5
K1
  Top 0.406: IC1.32 11.7,26.89 11.7,13.2 12.3,12.6 | UP.2 UP.1
  Top 0.508: 12.3,12.6 UP.2
K2  (via drill 0.5)
  Top 0.406: v22,14.2 SEL.2 SEL.1
  Top 0.508: IC1.1 14.22,25.02 v14.1,24.9
  Bottom 0.508: v14.1,24.9 22,17 v22,14.2
K3  (via drill 0.5)
  Top 0.406: v31.5,13.8 DWN.2 DWN.1
  Top 0.508: IC1.2 15.02,25.58 v15.6,25
  Bottom 0.508: v15.6,25 25.2,15.4 29.9,15.4 v31.5,13.8
KK
  Top 1.016: U1.8 39.91,49.4 L4.2 39.81,46.61 C7.1
MCLOSET
  Top 0.61: Q16.3 90.78,3.02 CLOSET.4
MFOOT1
  Top 0.61: Q12.3 88.58,33.6 FOOT1.4
MFOOT2
  Top 0.61: Q13.3 90.56,17.8 FOOT2.4
MISO
  Top 0.406: IC1.16 21.31,39.29 18.75,41.85 PROG.4
MOSI
  Top 0.406: PROG.3 22.6,41.33 22.6,34.6 23,34.2 23,33.3 22.42,32.72 IC1.15
MSTRIP
  Top 0.61: Q11.3 90.6,46.01 STRIP.4
N$1
  Top 0.508: 3.34,39.8 3.52,39.61 Q15.6 Q15.1 | J.2 4.11,40.56 Q15.5 Q15.2
  Top 1.016: R2.1 3.34,39.8 J.2
N$3
  Top 0.508: R1.2 12.6,48.8 Q21.E
N$4  (via drill 0.5)
  Top 0.406: R7.2 46.52,55.48 46.98,55.48 | 46.98,55.48 47.95,54.5 49.6,54.5 50.5,53.6 50.5,52.7 49.7,51.9 49.66,51.94 U1.3 | Q20.C 24.58,47.18 v24.6,47.2 | v30.7,47.2 R13.1 | 46.98,55.48 45.96,56.49 45.96,56.5 45.32,57.13 v45.1,57.13
  Bottom 0.406: v24.6,47.2 v30.7,47.2 32.6,49.1 32.6,51.7 38.03,57.13 v45.1,57.13
N$5
  Top 1.016: R5.2 R6.1 27.75,52.05 R4.1 25.3,54.7 R3.2
N$6
  Top 0.406: R17.2 82.74,55.05 Q1.E
N$7
  Top 0.406: MOF.3 44.15,55.6 R7.1
N$8
  Top 1.016: R2.2 3.4,34.59 3.2,34.39 PWR.1
N$9
  Top 0.406: R10.2 42.15,35.8 C2.1
N$10
  Top 0.406: R20.1 78.18,56.9 D7.2 78.56,56.95 Q1.B
N$11  (via drill 0.5)
  Top 0.406: U1.4 48.65,53.2 48.7,53.16 48.84,53.16 48.2,53.8 v46.6,53.8 | v39,39.3 37.8,38.1 C3.1 40.2,37.65 R10.1
  Bottom 0.406: v46.6,53.8 40.5,53.8 40,53.3 40,40.3 v39,39.3
N$12
  Top 0.508: Q20.B 24.69,49.9 29.5,49.9 30.66,51.06 R6.2
  Top 1.016: R4.2 30.66,54.64 R6.2 34.22,51.98 35.9,50.3 35.79,50.19 L4.1
N$13  (via drill 0.4)
  Top 0.406: R9.1 2.1,19.25 D2.C | R8.2 39.3,56.45 MOF.1
  Top 0.508: R8.2 35.65,56.45 v35.2,56 | v3.8,19.6 3.75,19.55 R9.1
  Bottom 0.508: v35.2,56 29.4,50.2 22.6,50.2 18.7,46.3 10.2,46.3 9.1,45.2 9.1,43.6 9.1,25.1 3.8,19.8 v3.8,19.6
N$16
  Top 0.508: R53.1 3.98,52.41 6.82,52.41 Q10.B 7.22,52.41 10.89,52.41 Q21.B | D1.C 3.52,56.48 3.52,54.11
  Top 1.016: R53.1 3.52,54.11 D22.A
N$19  (via drill 0.4)
  Top 0.406: R11.2 49.45,44.3 49.45,45.15 46.8,47.8 v43.4,47.8 | v41.5,52.2 42.51,53.2 U1.5
  Top 0.61: 49.45,44.3 R12.1
  Bottom 0.406: v43.4,47.8 41.5,49.7 v41.5,52.2
N$21
  Top 0.406: R18.2 82.66,51.83 Q2.E
N$23
  Top 0.406: R19.2 82.79,48.38 Q3.E
N$24
  Top 0.406: R21.1 74.45,52.95 74.98,53.48 78.25,53.48 D8.2 78.75,53.73 Q2.B
N$25
  Top 0.406: R22.1 73.92,49.02 74.9,50 78.25,50 D9.2 78.87,49.87 79.28,50.28 Q3.B
N$26
  Top 0.406: T3.3 71.11,55 R20.2
N$27
  Top 0.406: T4.3 71.12,51.05 R21.2
N$29
  Top 0.406: R23.2 64.34,56.21 R26.2 66.74,55.97 T3.1
N$30
  Top 0.406: T6.3 73.62,47.13 R22.2
N$31
  Top 0.406: R24.2 64.37,52.27 R27.2 68.66,52.27 T4.1
N$32
  Top 0.406: R25.2 R28.2 68.64,48.33 T6.1
N$33
  Top 0.406: R29.2 84.43,41.14 Q4.E
N$35
  Top 1.016: D22.C 8.52,54.28 D23.A
N$37
  Top 0.406: R30.2 84.32,37.96 Q5.E
N$39
  Top 0.406: R31.2 84.31,34.69 Q6.E
N$40
  Top 0.406: R32.1 77.6,43.35 D4.2 84.75,42.72 Q4.B
N$41
  Top 0.406: R33.1 73.65,39.46 78.06,39.46 D5.2 84.71,39.36 Q5.B
N$42
  Top 0.406: R34.1 74.24,36.16 D6.2 84.74,36.16 Q6.B
N$43
  Top 0.406: T5.3 73.56,41.47 R32.2
N$44
  Top 0.406: T7.3 73.46,33.48 R34.2
N$45
  Top 0.406: T8.3 73.53,37.56 R33.2
N$46
  Top 0.406: R35.2 66.36,42.55 R38.2 66.49,42.42 T5.1
N$47
  Top 0.406: R36.2 66.42,38.44 R39.2 68.72,38.37 T8.1
N$48
  Top 0.406: R37.2 66.38,34.28 R40.2 68.64,34.15 T7.1
N$49
  Top 0.406: R41.2 82.88,26.5 Q7.E
N$51
  Top 0.508: Q10.E 7.02,49.08 7.98,48.12 R54.2
N$53
  Top 0.406: R42.2 82.83,23.29 Q8.E
N$55
  Top 0.406: R43.2 84.55,20.55 Q9.E
N$56
  Top 0.406: R44.1 77.37,29.2 D30.2 84.92,28.51 Q7.B
N$57
  Top 0.406: R45.1 74.06,25.06 74.2,25.2 78.06,25.2 D31.2 84.94,25.11 Q8.B
N$58
  Top 0.406: R46.1 74.44,21.89 78.12,21.89 D32.2 78.31,21.96 Q9.B
N$59
  Top 0.406: T9.3 73.47,27.35 R44.2
N$60
  Top 0.406: T10.3 73.43,19.15 R46.2
N$61
  Top 0.406: T11.3 73.48,23.22 R45.2
N$62
  Top 0.406: R47.2 64.41,28.44 R50.2 66.82,28.3 T9.1
N$63
  Top 0.406: R48.2 66.7,24.21 R51.2 T11.1
N$64
  Top 0.406: R49.2 66.67,20.08 R52.2 68.8,20.07 T10.1
N$65  (via drill 0.4)
  Top 0.406: IC1.14 24.82,31.92 v26.2,33.3 | v29.8,35.7 31.3,35.7 v33.7,38.1 | v38.3,42.6 v41.4,42.6 | v80.5,46.4 80.52,46.42 R56.1 83.07,46.96 Q11.1
  Bottom 0.406: v26.2,33.3 28.6,35.7 v29.8,35.7 | v33.7,38.1 38.2,42.6 v38.3,42.6 | v41.4,42.6 48.7,42.6 51.1,45 79.1,45 v80.5,46.4
N$67  (via drill 0.4)
  Top 0.406: R57.1 79.94,32.44 79,31.5 79,31.1 v79.1,31 | v80.3,18.3 82.78,18.3 R58.1 84.02,18.21 84.55,18.75 Q13.1 | IC1.13 26.18,31.12 30,27.3 41.76,27.3 41.77,27.31 56.09,27.31 v56.3,27.1
  Top 0.61: R57.1 82.64,32.87 Q12.1
  Bottom 0.406: v79.1,31 79.1,19.5 v80.3,18.3 59.4,18.3 58.3,19.4 58.3,26.2 57.4,27.1 v56.3,27.1
N$71  (via drill 0.4)
  Top 0.406: IC1.12 25.38,30.32 29.4,26.3 v33.8,26.3 | v79.6,3.6 82.6,3.6 R59.1 84.58,3.57 Q16.1
  Bottom 0.406: v33.8,26.3 47.3,12.8 47.3,5 48.7,3.6 v79.6,3.6
N$72
  Top 0.406: R60.2 82.98,11.88 Q17.E
N$75
  Top 0.406: R61.2 84.48,9.32 Q18.E
N$77
  Top 0.406: R62.2 83.2,5.36 Q19.E
N$78
  Top 0.406: IC1.7 19.02,25.18 21.79,22.41 21.99,22.21 | 21.99,22.21 22,22.21 | 21.99,22.21 23.37,20.83 | 23.37,20.83 Q14.2 | C18.1 24.11,20.09 23.37,20.83
N$79
  Top 0.406: IC1.8 23.55,22.7 26.8,22.7 28.19,21.31 Q14.1 28.66,20.12 C19.1 28.26,17.2
N$80
  Top 0.406: R63.1 77.61,14.88 D10.2 78.06,14.8 84.06,14.8 Q17.B
N$81
  Top 0.406: R64.1 73.2,11.28 77.52,11.28 D11.2 78,10.8 84.9,10.8 Q18.B
N$82
  Top 0.406: R65.1 73.18,6.88 74,7.7 77.58,7.7 D12.2 84.76,7.55 Q19.B
N$83
  Top 0.406: T12.3 72.73,12.84 R63.2
N$84
  Top 0.406: T13.3 R65.2
N$85
  Top 0.406: T14.3 72.71,9.07 R64.2
N$87
  Top 0.406: R66.2 65.87,13.83 R69.2 67.52,13.82 67.7,14 67.91,13.79 T12.1
N$88
  Top 0.406: T14.1 67.97,9.86 R70.2 65.87,9.88 R67.2
N$89
  Top 0.406: T13.1 67.91,5.9 R71.2 65.82,5.99 R68.2
OCB
  Top 0.61: Q19.C 91.53,6.31 CLOSET.3
OCG
  Top 0.61: Q18.C 91.2,9.62 CLOSET.2
OCR
  Top 0.61: Q17.C 90.53,12.83 CLOSET.1
OFB1
  Top 0.61: Q6.C 88.8,35.2 89.74,36.14 FOOT1.3
OFB2
  Top 0.61: Q9.C 91.23,21.01 FOOT2.3
OFG1
  Top 0.61: Q5.C 91.51,38.46 FOOT1.2
OFG2
  Top 0.61: Q8.C 91.54,24.24 FOOT2.2
OFR1
  Top 0.61: Q4.C 91.24,41.71 FOOT1.1
OFR2
  Top 0.61: Q7.C 90.87,27.45 FOOT2.1
ONOFF
  Top 0.406: PWR.4 2.4,23.24 R9.2
OSB1
  Top 0.61: Q3.C 91.38,49.33 STRIP.3
OSG1
  Top 0.61: Q2.C 90.97,52.78 STRIP.2
OSR1
  Top 0.61: Q1.C 90.29,56 STRIP.1
OUT
  Top 0.61: U1.1 50.58,47.6 L3.1 51.89,50.89 D3.C
RESET
  Top 0.406: PROG.6 12.78,41.75 C17.1 12.76,39.4 11,39.4 10,38.4 10,31.1 10.78,30.32 IC1.29 | PROG.6 14.27,42.64 | PROG.6 15.43,44.4 16.6,44.4 17.51,45.31 R55.1
RX
  Top 0.406: IC1.30 11.52,29.52 8.6,26.6 8.6,21.2 4.4,17 4.4,12.5 6.01,10.89 HC-05.3
SB1  (via drill 0.4)
  Top 0.406: IC1.25 12.73,35.27 v12.7,35.3 | v30.5,37.8 33,40.3 45.6,40.3 46.7,41.4 56.9,41.4 62.54,47.04 R25.1
  Bottom 0.406: v12.7,35.3 14.7,37.3 30,37.3 v30.5,37.8
SCK
  Top 0.406: PROG.5 19.82,39.03 IC1.17
SG1  (via drill 0.4)
  Top 0.406: IC1.24 14.22,36.42 17.4,39.6 v17.5,39.6 | v30.5,42.1 32.2,43.8 v43.5,43.8 | v60.5,52.4 62.34,52.4 R24.1
  Bottom 0.406: v17.5,39.6 28,39.6 v30.5,42.1 | v43.5,43.8 52.1,52.4 v60.5,52.4
SR1  (via drill 0.4)
  Top 0.406: R23.1 61.63,56.23 v60.5,55.1 | v30.4,39.7 32,41.3 42.9,41.3 44.7,43.1 v44.7,46.8 | v18.6,38.4 17.4,38.4 15,36 15.02,35.98 IC1.23
  Bottom 0.406: v60.5,55.1 59.3,53.9 51.8,53.9 v44.7,46.8 | v30.4,39.7 29.1,38.4 23.7,38.4 v18.6,38.4
SUPOUT  (via drill 0.5, 0.7)
  Top 0.406: 78.1,9.08 79.9,9.08 | 79.9,9.08 80.21,9.08 | 75.68,12.28 76.58,12.28 77.02,12.71 D10.1 80.25,12.71 R60.1 | 75.73,8.73 76.53,8.73 76.88,9.08 78.1,9.08 | v75.9,5 77.08,5 D12.1 80,5.65 | v75.4,51.2 77.4,51.2 77.66,51.46 78.2,51.46 78.5,51.46 | 78.5,51.46 79.72,51.46 R18.1 | v76.1,47.1 77.52,47.1 D9.1 79.89,47.97 R19.1 | v75.6,54.5 78,54.5 D7.1 79.72,54.84 R17.1 | v76.9,33.2 76.99,33.2 D6.1 79.94,34.26 R31.1 | R30.1 79.87,37.45 D5.1 77.2,37.45 76.86,37.12 v76.1,37.12 | D4.1 80.18,40.82 R29.1 | 78.13,40.72 77.32,40.72 77,40.4 v76.3,40.4 | v76.4,19.5 77.75,19.5 D32.1 79.97,19.93 R43.1 | R41.1 80.28,26.61 D30.1 77.27,26.61 76.96,26.3 v76,26.3 | R42.1 78.58,23.64 D31.1 77.35,23.21 77.04,22.9 v76,22.9 | D8.1 78.5,51.46 | 79.9,9.08 80.14,9.32 R61.1 | 80,5.65 80.29,5.65 | R62.1 80.36,6.01 80,5.65 | D11.1 78.1,9.08 | C8.2 57.2,16.3
  Top 0.61: v75.7,8.7 75.73,8.73 | v75.66,12.3 75.68,12.28 | 78.13,40.72 D4.1 | v60.2,20.4 59.1,20.4 | 56.4,50.4 56.4,48.09 L3.2 55.91,44.46 | 56.4,50.4 C4.2 | 56.4,50.4 56.5,50.3 58.4,50.3 58.6,50.3 v60.7,50.3 | 55.91,44.46 R11.1 | 57.2,16.3 v59.1,16.3 59.1,20.4 | 59.1,20.4 57.5,22 C6.2 v56.7,24.8 | v54.1,31.1 56.7,33.7 v56.7,34.5 56.7,35.1 C5.2 v56.7,40 | v55.9,42.8 55.9,44.45 55.91,44.46
  Bottom 0.61: v75.9,5 75.59,5.31 75.59,8.69 75.6,8.7 v75.7,8.7 75.56,8.7 75.56,12.2 v75.66,12.3 71.66,16.3 v59.1,16.3 | v60.7,50.3 74.5,50.3 74.7,50.5 | 74.7,50.5 v75.4,51.2 | 74.7,50.5 74.7,48.3 75.9,47.1 v76.1,47.1 | 74.7,50.5 74.7,53.6 v75.6,54.5 | v56.7,34.5 75.7,34.5 | v76.9,33.2 75.7,34.4 75.7,34.5 | 75.7,34.5 75.7,36.72 | 75.7,36.72 v76.1,37.12 | 75.7,36.72 75.7,39.8 v76.3,40.4 | v60.2,20.4 75.5,20.4 | 75.5,20.4 v76.4,19.5 | 75.5,20.4 75.5,22.4 | 75.5,22.4 v76,22.9 | 75.5,22.4 75.5,25.8 v76,26.3 | v56.7,24.8 54.1,27.4 v54.1,31.1 | v56.7,40 56.7,42 v55.9,42.8
SUPPLY  (via drill 0.5, 0.65, 1)
  Top 0.305: Q21.C
  Top 0.406: Q20.E 21.3,48.41 v21.3,46.9 | v24.5,45.9 26.05,45.9 R13.2
  Top 0.508: 22.27,51.84 22.45,52.02 | v8.9,50.2 9.22,50.52 Q10.C | Q21.C 13.29,50.49 v13.1,50.3
  Top 0.61: 22.27,51.84 Q20.E 22.27,49.27
  Top 0.813: 3.36,45.03 TR1.P$2 | 3.31,47.31 C1.1 | Q15.4 4.54,42.66 J.1 3.36,43.2 4.8,43.2 5.69,42.31 Q15.4
  Top 1.016: TR1.P$2 3.36,45.14 C1.1 3.42,47.42 3.42,49.36 R53.2 | TR1.P$2 3.31,43.25 3.36,43.2 | v20.6,52 22.46,52 R5.1 22.45,52.02 R3.1 | v4.64,45.1 TR1.P$2
  Bottom 0.406: v24.5,45.9 22.3,45.9 v21.3,46.9
  Bottom 0.508: 7.14,48.3 8.9,50.05 v8.9,50.2 | v13.1,50.3 11.1,48.3 10.8,48.3
  Bottom 1.016: v20.6,52 20.6,50.6 18.3,48.3 10.8,48.3 7.14,48.3 6.64,48.3 | 6.64,48.3 4.64,46.3 v4.64,45.1 | 6.64,48.3
TX
  Top 0.406: IC1.31 11.87,28.72 10.39,27.24 10.39,15.89 7.93,13.43 HC-05.2
VCC  (via drill 0.4, 0.6)
  Top 0.406: IC1.20 17.42,33.68 17.8,33.3 v18.7,33.3 19.02,33.62 IC1.18 | C16.1 24.9,35.57 v24.9,34.1 | C15.2 16.6,22.61 | 16.6,22.61 18.3,22.61 | 18.3,22.61 18.51,22.61 C14.2 | IC1.6 18.22,22.69 18.3,22.61 | IC1.4 16.62,22.63 16.6,22.61 | 9.14,5.81 C20.1
  Top 0.508: v14.8,20.2 15.97,21.37 C15.2 | v3,10.5 3,8.72 R72.2 3.89,8.47 HC-05.5 9.14,5.81 | C12.1 14.7,52.81 C13.2 15.59,46.14 R55.2 15.58,46.15 R1.1 12.53,46.22 R54.1 | 10.5,45.78 v10.5,44.5 | C9.1 C20.1
  Top 0.61: R54.1 10.5,45.78
  Top 1.016: D23.C 14.62,54.25 C12.1
  Bottom 0.406: 10.5,35.6 10.5,35.5 11.9,34.1 17.9,34.1 v18.7,33.3 24.1,33.3 v24.9,34.1
  Bottom 0.508: v10.5,44.5 10.5,35.6 10.5,23.2 | 10.5,23.2 13.5,20.2 v14.8,20.2 | 10.5,23.2 7.8,20.5 4.3,17 4.3,11.8 v3,10.5
  Bottom 0.61: v10.5,44.5 24.51,44.5 PROG.1

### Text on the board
tPlace: R | R | G | B | M | M | LN-Electronic | R | R | G | B | + | M | M | - | R | R | G | ON/OFF | B | M | M | R | R | G | B | M | AMBIENT / CONTROLER V2 | M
